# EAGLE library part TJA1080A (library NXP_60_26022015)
FlexRay transceiver The TJA1080A is a FlexRay transceiver that is fully compliant with the FlexRay electrical physical layer specification V2.1 Rev. A. In addition, it incorporates features and parameters included in V3.0.1. It is primarily intended for communication systems from 1 Mbit/s to 10 Mbit/s, and provides an advanced interface between the protocol controller and the physical bus in a FlexRay network. The TJA1080A can be configured to be used as an active star transceiver or as a node transceiver. The TJA1080A provides differential transmit capability to the network and differential receive capability to the FlexRay controller. It offers excellent EMC performance as well as high ESD protection. The TJA1080A actively monitors the system performance using dedicated error and status information (readable by any microcontroller), as well as internal voltage and temperature monitoring. The TJA1080A supports the mode control as used in NXP Semiconductors TJA1054 and TJA1041 CAN transceivers. The TJA1080A is the next step up from the TJA1080 FlexRay transceiver. Being fully pin compatible and offering the same excellent ESD protection, the TJA1080A also features: Improved power-on reset concept Improved ElectroMagnetic Emission (EME) Support of 60 ns minimum bit time Improved bus error detection functionality This makes the TJA1080A an excellent choice in any kind of FlexRay node. See Section 14 for a detailed overview of differences between the TJA1080 and the TJA1080A.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
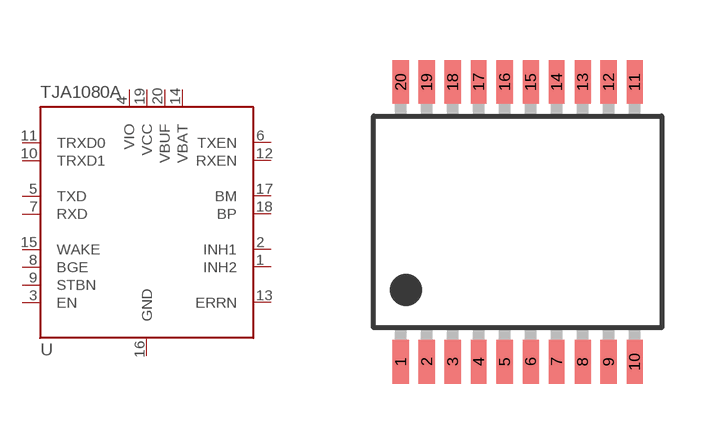
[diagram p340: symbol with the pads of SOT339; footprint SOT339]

Designator prefix U

## TJA1080ATS  [SOT339]
1  INH2  out
2  INH1  out
3  EN  in
4  VIO  pwr
5  TXD  in
6  TXEN  in
7  RXD  out
8  BGE  in
9  STBN  in
10  TRXD1
11  TRXD0
12  RXEN  out
13  ERRN  out
14  VBAT  pwr
15  WAKE  in
16  GND  pwr
17  BM
18  BP
19  VCC  pwr
20  VBUF  pwr

## Footprint SOT339 (pad centres in mm)
SOT339 SSOP20: plastic shrink small outline package; 20 leads; body width 5.3 mm JEDEC: MO-150 IEC: --
smd 0.4 x 1.1: 1 -2.925,-3.5; 2 -2.275,-3.5; 3 -1.625,-3.5; 4 -0.975,-3.5; 5 -0.325,-3.5; 6 0.325,-3.5; 7 0.975,-3.5; 8 1.625,-3.5; 9 2.275,-3.5; 10 2.925,-3.5; 11 2.925,3.5; 12 2.275,3.5; 13 1.625,3.5; 14 0.975,3.5; 15 0.325,3.5; 16 -0.325,3.5; 17 -0.975,3.5; 18 -1.625,3.5; 19 -2.275,3.5; 20 -2.925,3.5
